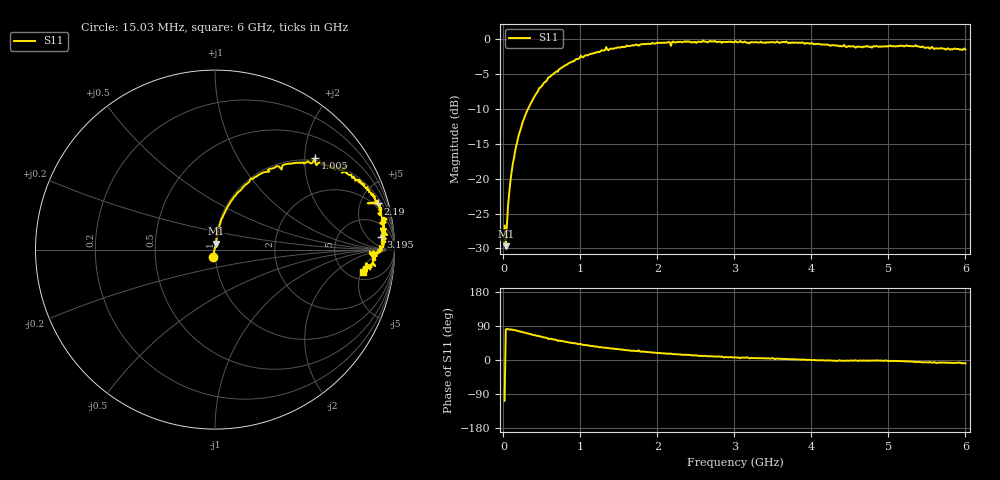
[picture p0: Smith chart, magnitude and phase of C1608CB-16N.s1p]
!	Network	Analyzer	HP8753E.07.74:	Oct	30	2002	Serial	No.	JP38451487
!	Hewlett-Packard
!	28	Aug	2009	7:55:30
!	Frequency	S11
#	HZ	S	RI	R	50
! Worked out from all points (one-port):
!   400 points, 15.03 MHz to 6 GHz, reference 50 ohm
!   lowest |S11| = -29.7 dB at 30.03 MHz (marker M1), VSWR 1.07, Z = 50.4 + j3.27 ohm
!   |S11| at or under -10 dB: start of sweep to 321.1 MHz
!   S11 on the Smith chart (normalised r, x): 15.03 MHz: 0.97, -0.09; 1.005 GHz: 0.94, +2.24; 2.19 GHz: 1.51, +6.86; 3.195 GHz: 14, +13; 6 GHz: 6.68, -5.46
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1.502992e7  -0.0139 -0.0439
3.002985e7  0.00544 0.0324
6.00297e7  0.00955 0.0635
1.050295e8  0.0189 0.109
1.650292e8  0.0347 0.167
2.550287e8  0.0752 0.247
4.650277e8  0.2 0.397
7.650262e8  0.4 0.477
1.005025e9  0.558 0.51
1.245024e9  0.667 0.443
1.335023e9  0.734 0.469
1.515022e9  0.763 0.4
1.725021e9  0.833 0.364
1.755021e9  0.801 0.387
1.785021e9  0.847 0.336
1.99502e9  0.89 0.294
2.160019e9  0.904 0.265
2.175019e9  0.851 0.258
2.190019e9  0.906 0.257
2.265019e9  0.918 0.247
3.015015e9  0.954 0.114
3.165014e9  0.924 0.119
3.195014e9  0.924 0.0686
3.765011e9  0.933 0.036
4.335008e9  0.888 -0.0426
4.515007e9  0.881 -0.0205
5.265004e9  0.885 -0.0602
6e9  0.827 -0.123
